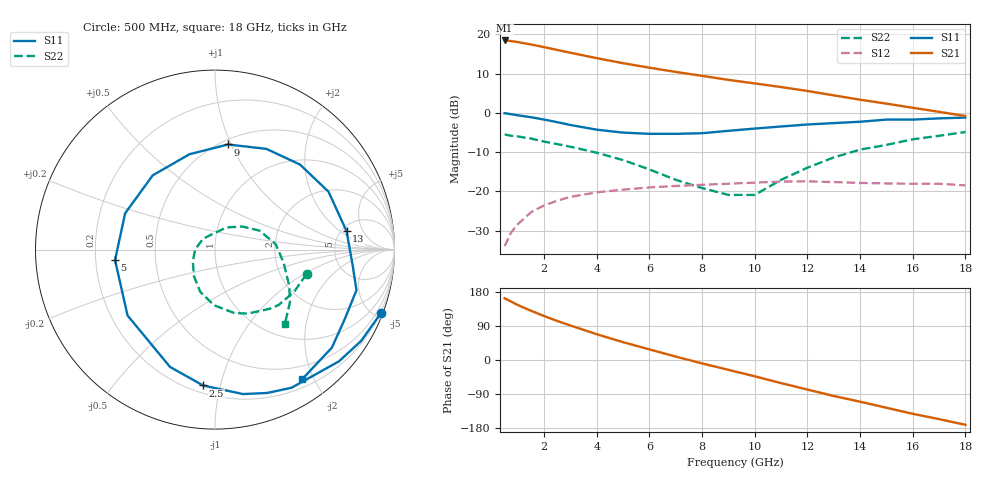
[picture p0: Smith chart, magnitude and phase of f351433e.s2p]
!ATF-35143
!S-PARAMETERS at Vds=3V  Id=30mA.  LAST UPDATED 06-3-99
# ghz s ma r 50
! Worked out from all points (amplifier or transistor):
!   23 points, 500 MHz to 18 GHz, reference 50 ohm
!   highest |S21| = 18.4 dB at 500 MHz (marker M1)
!   |S21| within 3 dB of that: start of sweep to 2.909 GHz
!   unconditionally stable (mu >= 1): 6.846 GHz to end of sweep
!   at 1.5 GHz: K = 0.31, MSG = 21.4 dB, |S12| = -25.4 dB
!   at 7 GHz: K = 1.01, MAG = 13.8 dB, |S12| = -18.6 dB
!   at 18 GHz: K = 1.24, MAG = 5.9 dB, |S12| = -18.5 dB
!   lowest NFmin = 0.11 dB at 500 MHz
!   S11 on the Smith chart (normalised r, x): 500 MHz: 0.15, -5.39; 2.5 GHz: 0.25, -0.89; 5 GHz: 0.28, -0.05; 9 GHz: 0.54, +0.97; 13 GHz: 5.52, +2.51; 18 GHz: 0.31, -1.84
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0.5  0.99 -21.0  8.36 163.0  0.02 77.0  0.53 -15.0
0.75  0.96 -32.0  8.21 154.0  0.03 70.0  0.51 -21.0
1  0.93 -42.0  7.97 145.0  0.038 65.0  0.5 -28.0
1.5  0.88 -61.0  7.43 130.0  0.054 54.0  0.47 -41.0
1.75  0.85 -70.0  7.15 123.0  0.06 50.0  0.45 -47.0
2  0.82 -79.0  6.87 116.0  0.066 45.0  0.43 -52.0
2.5  0.76 -95.0  6.33 103.0  0.076 37.0  0.4 -63.0
3  0.7 -111.0  5.83 91.0  0.085 29.0  0.37 -73.0
4  0.61 -143.0  4.97 68.0  0.097 15.0  0.31 -91.0
5  0.56 -174.0  4.29 47.0  0.105 2.0  0.25 -109.0
6  0.54 158.0  3.76 28.0  0.112 -10.0  0.19 -128.0
7  0.54 130.0  3.32 9.0  0.117 -22.0  0.14 -152.0
8  0.55 105.0  2.96 -9.0  0.121 -33.0  0.11 179.0
9  0.59 83.0  2.63 -26.0  0.125 -44.0  0.09 138.0
10  0.63 63.0  2.37 -43.0  0.129 -55.0  0.09 95.0
11  0.67 45.0  2.13 -61.0  0.133 -66.0  0.14 62.0
12  0.71 27.0  1.9 -78.0  0.134 -78.0  0.2 40.0
13  0.74 8.0  1.67 -95.0  0.131 -90.0  0.27 23.0
15  0.82 -16.0  1.31 -126.0  0.126 -110.0  0.39 -11.0
16  0.82 -28.0  1.16 -142.0  0.125 -120.0  0.46 -26.0
17  0.85 -40.0  1.03 -156.0  0.125 -131.0  0.51 -35.0
18  0.87 -56.0  0.91 -171.0  0.119 -142.0  0.57 -47.0
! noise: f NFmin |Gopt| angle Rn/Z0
0.5  0.11  0.87  4  0.18
0.9  0.16  0.81  13  0.17
1.5  0.23  0.72  26  0.16
1.8  0.27  0.68  33  0.15
2.5  0.35  0.59  49  0.14
3  0.41  0.53  63  0.12
5  0.66  0.37  123  0.07
6  0.79  0.33  157  0.05
8  1.04  0.31  -134  0.1
10  1.29  0.38  -68  0.28
